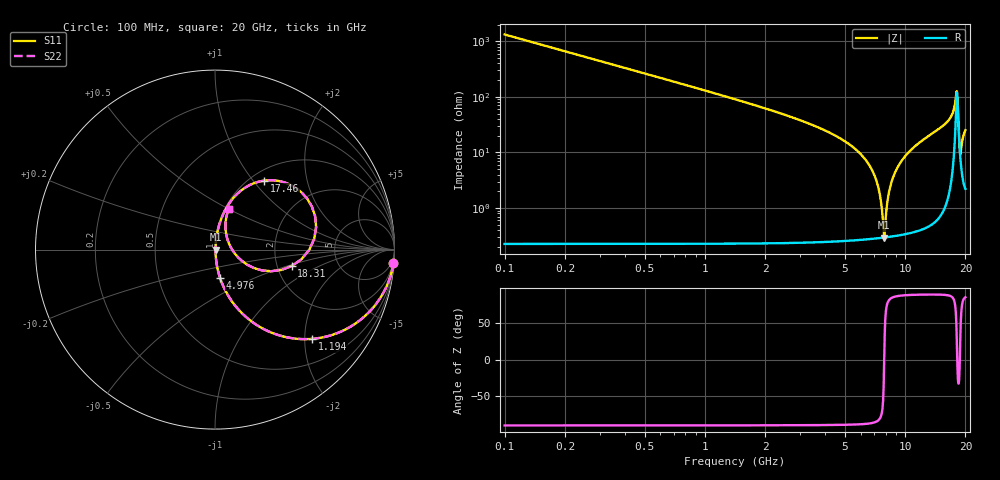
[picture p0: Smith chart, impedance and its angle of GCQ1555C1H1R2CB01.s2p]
!Murata Part Number: GCQ1555C1H1R2CB01
!These Parameters are Measured in Series Mode Connection
!Data Generated on Mar 13, 2026
!  o--ll--o
!Port1  Port2
!  o------o
!Operation Temp=25[degC], DC Bias Voltage=0[V]
!Freq. Start=100[MHz] Stop=20[GHz] 401[Steps]
# Hz S RI R 50
!Freq.(Hz) S11(Real) S11(Imag) S21(Real) S21(Imag) S12(Real) S12(Imag) S22(Real) S22(Imag)
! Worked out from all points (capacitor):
!   401 points, 100 MHz to 20 GHz, reference 50 ohm
!   read as one part in series: C = 1.2 pF near 199.5 MHz
!   lowest |Z| = 295 mohm at 7.861 GHz (marker M1)
!   series resonance near 7.863 GHz, so ESL is about 340 pH
!   S11 on the Smith chart (normalised r, x): 100 MHz: 1, -27; 1.194 GHz: 1.00, -2.17; 4.976 GHz: 1.01, -0.32; 17.46 GHz: 1.15, +1.14; 18.31 GHz: 2.40, -0.55; 20 GHz: 1.04, +0.50
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1e8  0.9943 -0.075  0.00567 0.075  0.00567 0.075  0.9943 -0.075
4.98e8  0.8754 -0.3299  0.1246 0.3299  0.1246 0.3299  0.8754 -0.3299
1.1945e9  0.5407 -0.4973  0.4593 0.4973  0.4593 0.4973  0.5407 -0.4973
2.13975e9  0.2492 -0.4305  0.7508 0.4305  0.7508 0.4305  0.2492 -0.4305
3.43325e9  0.0915 -0.2845  0.9085 0.2845  0.9085 0.2845  0.0915 -0.2845
4.9755e9  0.0277 -0.1563  0.9723 0.1563  0.9723 0.1563  0.0277 -0.1563
6.7665e9  0.00542 -0.0513  0.9946 0.0513  0.9946 0.0513  0.00542 -0.0513
7.41325e9  0.00328 -0.0202  0.9967 0.0202  0.9967 0.0202  0.00328 -0.0202
7.861e9  0.00294 -9.46e-05  0.9971 9.46e-05  0.9971 9.46e-05  0.00294 -9.46e-05
8.20925e9  0.00322 0.0148  0.9968 -0.0148  0.9968 -0.0148  0.00322 0.0148
8.5575e9  0.00392 0.0292  0.9961 -0.0292  0.9961 -0.0292  0.00392 0.0292
1.005e10  0.0109 0.0861  0.9891 -0.0861  0.9891 -0.0861  0.0109 0.0861
1.338325e10  0.0462 0.1985  0.9538 -0.1985  0.9538 -0.1985  0.0462 0.1985
1.67165e10  0.1542 0.3359  0.8458 -0.3359  0.8458 -0.3359  0.1542 0.3359
1.746275e10  0.2738 0.3843  0.7262 -0.3843  0.7262 -0.3843  0.2738 0.3843
1.79105e10  0.4842 0.3169  0.5158 -0.3169  0.5158 -0.3169  0.4842 0.3169
1.81095e10  0.5634 0.1259  0.4366 -0.1259  0.4366 -0.1259  0.5634 0.1259
1.83085e10  0.4272 -0.092  0.5728 0.092  0.5728 0.092  0.4272 -0.092
1.855725e10  0.1802 -0.0844  0.8198 0.0844  0.8198 0.0844  0.1802 -0.0844
1.885575e10  0.0772 0.0352  0.9228 -0.0352  0.9228 -0.0352  0.0772 0.0352
1.9403e10  0.0599 0.161  0.9401 -0.161  0.9401 -0.161  0.0599 0.161
2e10  0.0774 0.2266  0.9226 -0.2266  0.9226 -0.2266  0.0774 0.2266
